(* Logix 5000 AddOnInstructionDefinition export MSQE_Yaskawa; software revision 17.00 *)

TYPE Yaskawa_EIP_Servo :   // Yaskawa SigmaLogic Axis Structure v2.4.0
STRUCT
   O : Yaskawa_OUT_to_Servo;
   I : Yaskawa_IN_from_Servo;
   AOI_SB : Yaskawa_AOI_Status_Bits;
END_STRUCT
END_TYPE

TYPE Yaskawa_OUT_to_Servo :   // Structure of data sent out to the Yaskawa SigmaLogic controller v2.4.0
STRUCT
   b00_ServoOn : BOOL;   // Servo On
   b01_Stop : BOOL;   // Stops All Current Motion in Progress
   b02_Home : BOOL;   // Start Homing Process
   b03_MoveStart1 : BOOL;   // Start Current Motion
   b06_SuperImpose : BOOL;
   b07_ServoAlarmReset : BOOL;   // Servo Alarm Reset
   b08_ControllerAlarmReset : BOOL;   // SigmaLogic Alarm Reset
   b09_MoveStart2 : BOOL;   // Start Second Motion (Blended Move)
   b10_MoveAbort : BOOL;   // Abort Current Move
   b11_MovePause : BOOL;   // Pause Current Move
   b12_SeqPause : BOOL;   // Indexing Sequence Pause
   b13_SeqResume : BOOL;   // Indexing Sequence Resume
   b14_SeqCancel : BOOL;   // Indexing Sequence Cancel
   b15_AbsEncoderReset : BOOL;   // Absolute Encoder Reset
   b16_SeqStart : BOOL;   // Start Indexing Sequence
   b17_SeqEditSpeed : BOOL;   // Enter Edit Speed
   b18_SeqEditDistance : BOOL;   // Enter Distance Edit
   b19_PLSEnable : BOOL;   // Enable PLS execution
   b20_PLSActivateOutput1 : BOOL;   // Activate PLS output1 switch logic
   b21_PLSActivateOutput2 : BOOL;   // Activate PLS output2 switch logic
   b22_PLSActivateOutput3 : BOOL;   // Activate PLS output3 switch logic
   b23_PLSActivateOutput4 : BOOL;   // Activate PLS output4 switch logic
   b24_SetClock : BOOL;   // Set the remote controller clock with data provided by the PLC
   RebootController : BOOL;
   UseExternalEncoder : BOOL;   // Use External Encoder when executing MAHSP_Yaskawa
   b32_HeatbeatAnswer : BOOL;   // Heartbeat Answer
   BrakeBypassRequest : BOOL;
   SetFwdTorqueLimit : BOOL;
   SetRevTorqueLimit : BOOL;
   TorqueLimit : DINT;
   TorqueRamp : DINT;
   HomeMethod : INT;
   HomeSpeed : DINT;
   HomeAccDec : DINT;   // Home Move Acceleration/Deceleration Rate
   HomeBackOffDistance : DINT;
   HomeCreepSpeed : DINT;
   HomeCreepDistanceLimit : DINT;
   HomeCreepTimeLimit : DINT;
   HomeOffsetDistance : DINT;
   HomeOffsetSpeed : DINT;
   HomePostion : DINT;
   HomeTorque : DINT;
   HomeInputNo : DINT;
   HomeApproachTimeLimit : DINT;
   HomeApproachDistLimit : DINT;
   HomeDirection : INT;
   HomeSwitchMode : INT;
   MoveType : INT;
   MoveDirection : INT;
   MoveAccel1 : DINT;
   MoveAccel2 : DINT;
   MoveDecel1 : DINT;
   MoveDecel2 : DINT;
   MoveSpeed1 : DINT;
   MoveSpeed2 : DINT;
   MoveDistance1 : DINT;
   MoveDistance2 : DINT;
   MovePosition1 : DINT;
   MovePosition2 : DINT;
   RegistrationDistance : DINT;
   GearNumerator : DINT;
   GearDenominator : DINT;
   SuperImposeDistance : DINT;
   Resolution : INT;
   RegistrationDirection : INT;
   TuningLevel : INT;
   SequenceStep : INT;   // Staring Sequence Step Number
   SequenceEditStep : INT;   // Sequence Step Number to Edit
   FlagCommandBits1 : DINT;   // Flag Commands. 1..64 are General Flags, Bits 0..31 correspond to Flag 1..32
   FlagCommandBits2 : DINT;   // Flag Commands cont. 1..64 are General Flags, Bits 0..31 correspond to Flag 33..64
   DigitalOutCommandBits : DINT;   // Digital Output commands. Bits 0-7 correspond to CN13 Digital Outputs 0-7, used as Flag 73-80. Bits 8-10 correspond to CN1 Digital Outputs 0-2 used as Flag 88-90"
   SequenceEditSpeed : DINT;
   SequenceEditDistance : DINT;
   FeedRateOverride : INT;
   HSI_Enable : BOOL;
   HSI_MoveMode : BOOL;   // 0=Relative; 1=Moves per Cycle
   HSI_CalcMethod : BOOL;   // 0=Accel/Decel; 1=Time
   HSI_MoveDirection : BOOL;   // 0 = Negative; 1 = Positive
   HSI_TriggerFlag : INT;
   HSI_MovingFlag : INT;
   HSI_DwellingFlag : INT;
   HSI_DoneFlag : INT;
   HSI_MoveType : INT;   // 0=Single; 1=Repeat; 2=Repeat "x" times
   HSI_RepeatNumber : INT;
   HSI_Distance : DINT;
   HSI_Speed : DINT;
   HSI_Accel : DINT;
   HSI_MoveTime : DINT;
   HSI_DwellTime : DINT;
   PLS_OutputFlag1 : INT;
   PLS_OutputFlag2 : INT;
   PLS_OutputFlag3 : INT;
   PLS_OutputFlag4 : INT;
   PLS_OnPosition1 : DINT;
   PLS_OffPosition1 : DINT;
   PLS_OnPosition2 : DINT;
   PLS_OffPosition2 : DINT;
   PLS_OnPosition3 : DINT;
   PLS_OffPosition3 : DINT;
   PLS_OnPosition4 : DINT;
   PLS_OffPosition4 : DINT;
   PLS_OnCompensation1 : INT;
   PLS_OffCompensation1 : INT;
   PLS_OnCompensation2 : INT;
   PLS_OffCompensation2 : INT;
   PLS_OnCompensation3 : INT;
   PLS_OffCompensation3 : INT;
   PLS_OnCompensation4 : INT;
   PLS_OffCompensation4 : INT;
   RTC_Year : INT;
   RTC_Month : INT;
   RTC_Day : INT;
   RTC_Hour : INT;
   RTC_Min : INT;
   RTC_Sec : INT;
   StopDecel : DINT;
   AnalogOutput : INT;   // CN13, AO_01 [mV]
END_STRUCT
END_TYPE

TYPE Yaskawa_AOI_Status_Bits :   // Internal bits used to interlock Yaskawa AOI execution. v2.4.0
STRUCT
   MAM : BOOL;   // Move AOI Active
   MAJ : BOOL;   // Jog AOI Active
   MAB : BOOL;   // Blending AOI Active
   MAG : BOOL;   // Gearing AOI Active
   MAHSP : BOOL;   // Home SetPoint AOI Active
   MAH : BOOL;   // Homing AOI Active
   MSQE : BOOL;   // Sequence Edit AOI Active
   MSQR : BOOL;   // Sequence Run AOI Active
   MHSI : BOOL;   // High Speed Index AOI Active
   MSO : BOOL;   // Servo On
   MSF : BOOL;   // Servo Off
   MAFR : BOOL;   // Fault Reset
   MAS : BOOL;   // Servo Abort
   MTRQ : BOOL;   // Torque Mode Active
   MPLS : BOOL;   // PLS Active
   MCLK : BOOL;   // SetClock Active
   MSTL : BOOL;   // Set Torque Limit Active
   AOI_Permissive : BOOL;   // Permissive to Execute an AOI
END_STRUCT
END_TYPE

TYPE Yaskawa_IN_from_Servo :   // Structure of data coming from the Yaskawa SigmaLogic controller. v2.4.0
STRUCT
   AlarmText : STRING;   // ServoPack Alarm Code plus Text Description
   b00_Heartbeat : BOOL;
   b01_Alarm : BOOL;   // ServoPack Alarm
   b02_Warning : BOOL;   // ServoPack Warning
   b03_Ready : BOOL;   // ServoPack Ready
   b04_Enabled : BOOL;   // ServoPack Enabled ("Servo On")
   b05_StopComplete : BOOL;
   b06_HomeComplete : BOOL;
   b07_HomeBusy : BOOL;
   b08_HomeActive : BOOL;
   b09_HomeAborted : BOOL;
   b10_HomeError : BOOL;
   b11_MoveAbsComplete : BOOL;
   b12_MoveAbsBusy : BOOL;
   b13_MoveAbsActive : BOOL;
   b14_MoveAbsAborted : BOOL;
   b15_MoveAbsError : BOOL;
   b16_MoveRelComplete : BOOL;
   b17_MoveRelBusy : BOOL;
   b18_MoveRelActive : BOOL;
   b19_MoveRelAborted : BOOL;
   b20_MoveRelError : BOOL;
   b21_JogAtSpeed : BOOL;
   b22_JogBusy : BOOL;
   b23_JogActive : BOOL;
   b24_JogAborted : BOOL;
   b25_JogError : BOOL;
   b26_GearInSync : BOOL;
   b27_GearBusy : BOOL;
   b28_GearActive : BOOL;
   b29_GearAborted : BOOL;
   b30_GearError : BOOL;
   b32_MoveSuperComplete : BOOL;
   b33_MoveSuperBusy : BOOL;
   b34_MoveSuperActive : BOOL;
   b35_MoveSuperAborted : BOOL;
   b36_MoveSuperError : BOOL;
   b37_PowerCycleRequired : BOOL;
   b38_MoveBlend1Complete : BOOL;
   b39_MoveBlend1Busy : BOOL;
   b40_MoveBlend1Active : BOOL;
   b41_MoveBlend1Abort : BOOL;
   b42_MoveBlend1Error : BOOL;
   b43_MoveBlend2Complete : BOOL;
   b44_MoveBlend2Busy : BOOL;
   b45_MoveBlend2Active : BOOL;
   b46_MoveBlend2Abort : BOOL;
   b47_MoveBlend2Error : BOOL;
   b48_RegComplete : BOOL;
   b49_RegBusy : BOOL;
   b50_RegActive : BOOL;
   b51_RegAborted : BOOL;
   b52_RegError : BOOL;
   b53_ResetAbsEncoderActive : BOOL;
   b54_ResetAbsEncoderBusy : BOOL;
   b55_ResetAbsEncoderDone : BOOL;
   b56_ResetAbsEncoderError : BOOL;
   b57_SeqRunning : BOOL;
   b58_RegSensorNotReached : BOOL;
   b59_SeqEditError : BOOL;
   b60_SeqEditDone : BOOL;
   b61_TorqueAtTorque : BOOL;
   b62_TorqueBusy : BOOL;
   b63_TorqueActive : BOOL;
   b64_TorqueAborted : BOOL;
   b65_TorqueError : BOOL;
   b66_ControllerAlarm : BOOL;
   b67_ApplicationError : BOOL;
   b68_AxisAtStandStill : BOOL;
   b69_TestModeActive : BOOL;
   b70_ServoParamsOK : BOOL;
   b71_SetFwdTorqueLimitDone : BOOL;
   b72_SetRevTorqueLimitDone : BOOL;
   Position : DINT;
   Speed : DINT;
   Torque : DINT;
   HomeErrorID : INT;
   MoveAbsErrorID : INT;
   MoveRelErrorID : INT;
   JogErrorID : INT;
   GearErrorID : INT;
   MoveSuperErrorID : INT;
   ServoAlarmID : INT;
   ServoWarningID : INT;
   ControllerAlarmID : DINT;
   AxisGenAlarmID : DINT;
   MoveBlend1ErrorID : INT;
   MoveBlend2ErrorID : INT;
   ResetAbsEncoderErrorID : INT;
   FunctionBlockErrorID : INT;
   TorqueErrorID : INT;
   RegErrorID : INT;
   SeqCurrentStep : INT;
   FlagStatusBit1 : DINT;   // Flag Status. 1..64 are General Flags, Bits 0..31 correspond to Flag 1..32
   FlagStatusBit2 : DINT;   // Flag Status cont. 1..64 are General Flags, Bits 0..31 correspond to Flag 33..64
   IOStatusBits : DINT;   // Digital IO Status. Bits 0-7, CN13 Inputs 0-7, Used as Flag 65-72. Bits 8-15, CN13 Outputs 0-7, Used as Flag 73-80. Bits 16-22, CN1 Inputs 0-6, Used as Flag 81-87. Bits 23-25, CN1 Outputs 0-4, Used as Flag 88-92.
   HSI_Moving : BOOL;
   HSI_Dwelling : BOOL;
   HSI_Done : BOOL;
   HSI_Busy : BOOL;
   HSI_Error : BOOL;
   HSI_ErrorCode : INT;
   PLS_Running : BOOL;
   PLS_SwitchStatus1 : BOOL;
   PLS_SwitchStatus2 : BOOL;
   PLS_SwitchStatus3 : BOOL;
   PLS_SwitchStatus4 : BOOL;
   PLS_Busy : BOOL;
   PLS_Error : BOOL;
   PLS_ErrorCode : INT;
   SetClock_Done : BOOL;
   SetClock_Busy : BOOL;
   SetClock_Error : BOOL;
   SetClock_ErrorID : INT;
   SoftwareVersion : DINT;
   FirmwareVersion : DINT;
   CommandedPos : DINT;
   CommandedPosNonCyc : DINT;
   CommandedSpeed : DINT;
   Clock_Year : INT;
   Clock_Month : INT;
   Clock_Day : INT;
   Clock_Hour : INT;
   Clock_Minute : INT;
   Clock_Second : INT;
   AnalogInput : REAL;   // CN13, AI_01 [v]
   BrakeBypassActive : BOOL;
   ForwardTorqueLimit : DINT;
   ReverseTorqueLimit : DINT;
END_STRUCT
END_TYPE

ADD_ON_INSTRUCTION MSQE_Yaskawa   (* revision 2.4 0, vendor Yaskawa America, Inc., ExecuteEnableInFalse *)
// Motion Sequence Edit
// Revision note:
// 2.4.0: No functional change
// 2.3.1: No functional change
// 2.3.0: No functional change
// 2.0.0: No functional change.
// 1.2.0: No functional change.
// Initial Release 9/10/2014
// Help:
// This AOI edits the speed or distance parameter of a step in the predefined Sequence Table. This change is only made in RAM. When the controller is warm started or rebooted, the step parameters will revert back to the values transferred in from the LogicWorks Configuration Utility file.
// Sequence steps may not be edited while executing.
VAR_IN_OUT
   Axis : Yaskawa_EIP_Servo; {required}
END_VAR
VAR_INPUT
   SeqEditType : INT; {required}   // 1 = Edit Speed 2 = Edit Distance 3 = Edit Both
   SeqEditStepNo : INT; {required}   // Sequence Step # to Edit (Range is 1 to 200)
   SeqEditSpeed : REAL; {required}   // The new Speed for the given Step #
   SeqEditDistance : REAL; {required}   // The new Distance for the given Step #
END_VAR
VAR_OUTPUT
   EN : BOOL; {visible}   // Function is executing
   DN : BOOL; {visible}   // Sequence Edit Completed
   ER : BOOL; {visible}   // Sequence Edit Error
   FLT_BSY : BOOL; {visible}   // There is another AOI Active for this Axis
END_VAR
VAR
   AOI_ON_LOCAL : BOOL;
   ScaleFactor : INT;
   Seq_ER : BOOL;
END_VAR

ROUTINE EnableInFalse   (* ladder *)
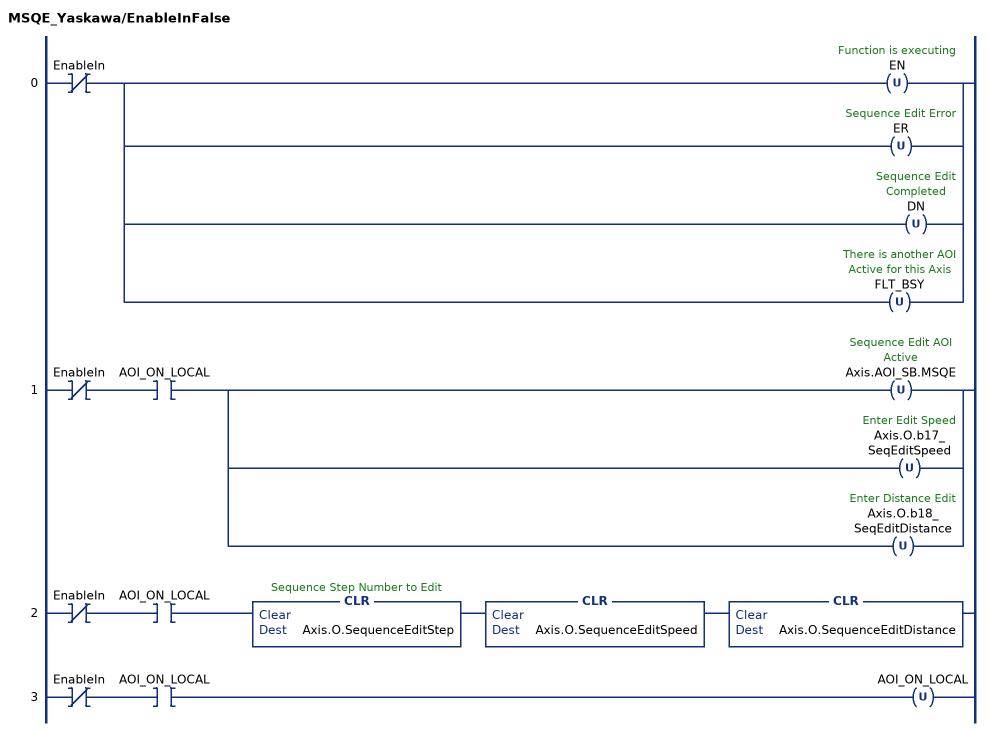
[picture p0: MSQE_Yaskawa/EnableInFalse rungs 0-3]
   0: XIO(EnableIn)[OTU(EN) ,OTU(ER) ,OTU(DN) ,OTU(FLT_BSY) ];
   1: XIO(EnableIn)XIC(AOI_ON_LOCAL)[OTU(Axis.AOI_SB.MSQE) ,OTU(Axis.O.b17_SeqEditSpeed) ,OTU(Axis.O.b18_SeqEditDistance) ];
   2: XIO(EnableIn)XIC(AOI_ON_LOCAL)CLR(Axis.O.SequenceEditStep)CLR(Axis.O.SequenceEditSpeed)CLR(Axis.O.SequenceEditDistance);
   3: XIO(EnableIn)XIC(AOI_ON_LOCAL)OTU(AOI_ON_LOCAL);
END_ROUTINE

ROUTINE Logic   (* ladder *)
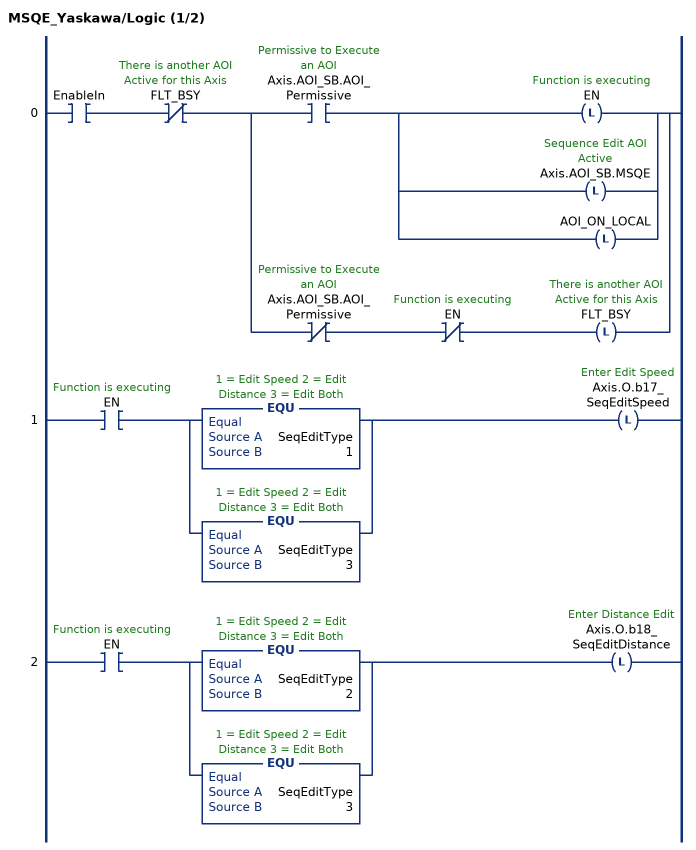
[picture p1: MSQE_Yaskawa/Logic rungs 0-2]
   0: XIC(EnableIn)XIO(FLT_BSY)[XIC(Axis.AOI_SB.AOI_Permissive) [OTL(EN) ,OTL(Axis.AOI_SB.MSQE) ,OTL(AOI_ON_LOCAL) ] ,XIO(Axis.AOI_SB.AOI_Permissive) XIO(EN) OTL(FLT_BSY) ];
   1: XIC(EN)[EQU(SeqEditType,1) ,EQU(SeqEditType,3) ]OTL(Axis.O.b17_SeqEditSpeed);
   2: XIC(EN)[EQU(SeqEditType,2) ,EQU(SeqEditType,3) ]OTL(Axis.O.b18_SeqEditDistance);
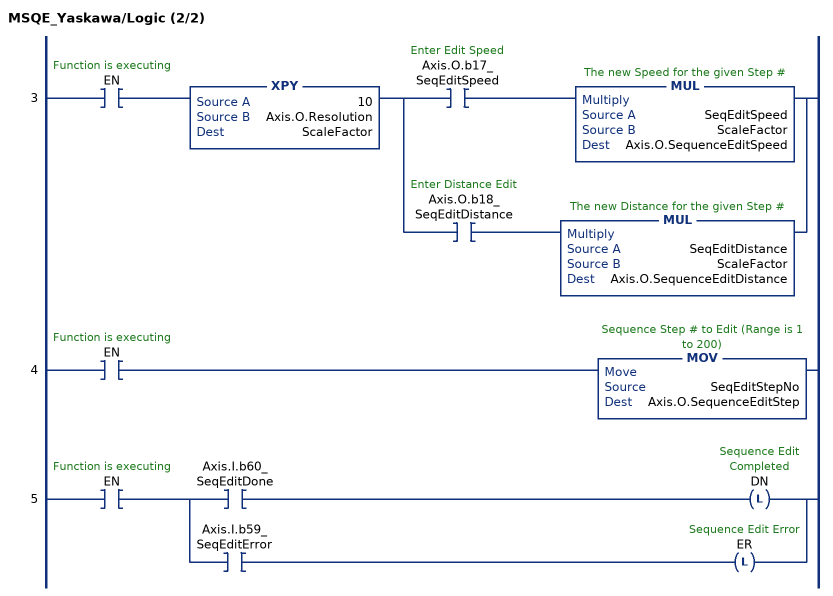
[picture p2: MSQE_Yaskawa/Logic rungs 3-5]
   3: XIC(EN)XPY(10,Axis.O.Resolution,ScaleFactor)[XIC(Axis.O.b17_SeqEditSpeed) MUL(SeqEditSpeed,ScaleFactor,Axis.O.SequenceEditSpeed) ,XIC(Axis.O.b18_SeqEditDistance) MUL(SeqEditDistance,ScaleFactor,Axis.O.SequenceEditDistance) ];
   4: XIC(EN)MOV(SeqEditStepNo,Axis.O.SequenceEditStep);
   5: XIC(EN)[XIC(Axis.I.b60_SeqEditDone) OTL(DN) ,XIC(Axis.I.b59_SeqEditError) OTL(ER) ];
END_ROUTINE
END_ADD_ON_INSTRUCTION
